
FUNCTION_BLOCK FB6

TITLE =   <Control de arranque motor diesel>
//
//
//
//
//
//
//

AUTHOR:   H3       //  Hedgar Hernandez H.
FAMILY:   CAT      //  Caterpillar 3616
NAME:     C3616    //
VERSION:  01.01    //  Version Inicial 25/01/2009
// KNOW_HOW_PROTECT

//
//
//
//
//
//
//

VAR_INPUT

  MODO_REMOTO  : BOOL;	  // Selector en Modo remoto.
  ARRANQUE_REM : BOOL;    // Peticion de arranque remoto.
  PARO_REM     : BOOL;    // Peticion de paro remoto.
  REM_LISTO	   : BOOL;    // Condiciones para arranque en remoto ok.
  PARO_MAQUINA : BOOL;    // Paro de maquina por falla mayor.
  DIESEL_OP    : BOOL;    // Motor Diesel operando.
  TI_MARCHA    : TIME;    // Tiempo de marcha al motor.
  P_ARR_LISTA  : BOOL;    // Presion de prelubricacion lista.
  RESET        : BOOL;    // Reset de fallas.
  DIESEL_RPM   : REAL;    // Velocidad de la maquina diesel RPM.

END_VAR


//VAR_IN_OUT

  // NUM_INTENTOS : INT;	  // Numero de intentos de arranque en modo automatico remoto.

//END_VAR


VAR_OUTPUT
  VAL_ARRANQUE    : BOOL;	// Salida a valvula de Arranque.
  VAL_COMBUSTIBLE : BOOL;   // Valvula de corte de Combustible.
  VAL_AIRE        : BOOL; 	// Valvula de corte de Aire.
  BOMBA_PRELUB	  : BOOL;   // Bomba de prelubricacion.
  TORRETA		  : BOOL;   // Torreta para aviso de arranque.
  F_ARR_REM		  : BOOL;   // Falla de arranque remoto.
END_VAR

VAR
  TEMP1, TEMP2, TEMP3, TEMP4 : TON;

END_VAR

// VAR_TEMP
//  ;
// END_VAR

BEGIN
NETWORK
TITLE =   <Recepcion de comandos remotos>
//
//
//
//


END_FUNCTION_BLOCK


